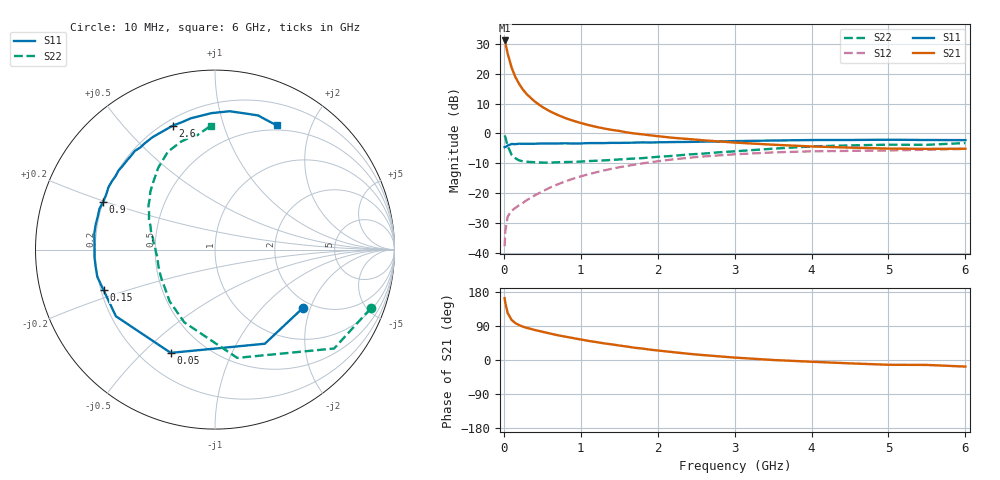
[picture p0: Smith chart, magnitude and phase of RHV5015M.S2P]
! SIEMENS Small Signal Semiconductors
! BFR106
! Si NPN RF Bipolar Junction Transistor in SOT23
! VCE = 0.5 V  IC = 15 mA
! Common Emitter S-Parameters:  August  1996
# GHz  S  MA  R  50
!  f  S11  S21  S12  S22
! GHz  MAG  ANG  MAG  ANG  MAG  ANG  MAG  ANG
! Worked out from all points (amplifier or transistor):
!   36 points, 10 MHz to 6 GHz, reference 50 ohm
!   highest |S21| = 31.2 dB at 10 MHz (marker M1)
!   |S21| within 3 dB of that: start of sweep to 38 MHz
!   unconditionally stable (mu >= 1): 355.8 MHz to end of sweep
!   at 250 MHz: K = 0.87, MSG = 19.0 dB, |S12| = -23.3 dB
!   at 1.4 GHz: K = 1.12, MAG = 4.5 dB, |S12| = -11.9 dB
!   at 6 GHz: K = 1.03, MAG = -1.0 dB, |S12| = -5.2 dB
!   S11 on the Smith chart (normalised r, x): 10 MHz: 1.79, -1.78; 50 MHz: 0.32, -0.61; 150 MHz: 0.21, -0.17; 900 MHz: 0.20, +0.19; 2.6 GHz: 0.23, +0.69; 6 GHz: 0.44, +1.52
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0.01  0.5878 -33.6  36.43 163.4  0.0128 77.5  0.9272 -20.7
0.02  0.5934 -62.1  32.91 149.9  0.0236 65.0  0.8626 -39.7
0.05  0.626 -113.2  21.93 123.7  0.0402 46.2  0.6159 -78.4
0.1  0.6653 -146.1  12.85 105.9  0.0502 39.2  0.4398 -112.9
0.15  0.6606 -159.9  8.836 97.3  0.0562 40.7  0.3834 -131.3
0.2  0.6731 -167.1  6.756 92.0  0.0624 43.5  0.3522 -142.3
0.25  0.6718 -172.7  5.407 87.8  0.0685 46.1  0.3402 -150.8
0.3  0.6726 -176.3  4.541 84.8  0.0761 49.3  0.3346 -155.9
0.4  0.6723 177.1  3.451 79.3  0.091 53.0  0.3282 -164.0
0.5  0.6785 172.4  2.788 74.6  0.1064 55.0  0.3248 -169.5
0.6  0.6793 168.1  2.349 69.9  0.1233 56.3  0.324 -173.0
0.7  0.6789 163.9  2.047 65.3  0.1397 56.6  0.328 -176.2
0.9  0.6777 157.1  1.637 57.8  0.1736 56.0  0.3327 177.8
1.1  0.688 149.7  1.384 50.5  0.2067 54.4  0.3438 173.9
1.3  0.6887 143.5  1.213 44.0  0.2392 51.8  0.3524 169.3
1.6  0.6978 134.8  1.04 35.4  0.2852 47.6  0.3728 163.4
2.2  0.7166 119.0  0.845 20.7  0.3665 37.8  0.4203 150.9
2.6  0.7296 108.7  0.766 12.8  0.4108 31.1  0.4591 142.5
3.5  0.7605 91.5  0.647 0.0  0.4803 16.7  0.5547 124.8
4.5  0.7766 77.8  0.578 -8.9  0.5102 3.0  0.6307 107.4
5.5  0.7757 67.5  0.551 -13.0  0.5333 -5.1  0.6447 98.9
6  0.7733 63.6  0.554 -17.4  0.5483 -11.3  0.6899 92.0
